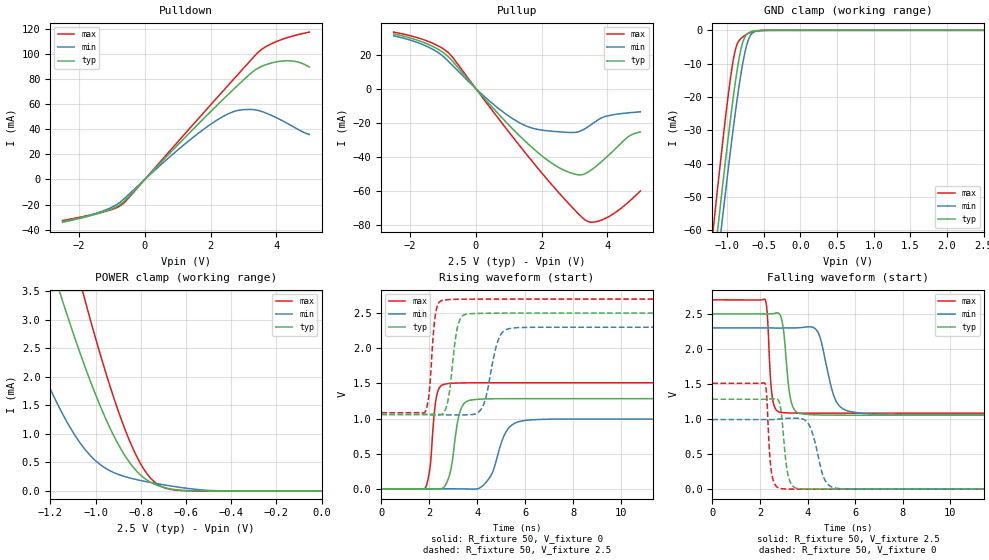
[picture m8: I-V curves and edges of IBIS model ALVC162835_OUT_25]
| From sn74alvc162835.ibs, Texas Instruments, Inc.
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[Model]   ALVC162835_OUT_25
Model_type  3-state
Enable   Active-Low
Vref =   0
Rref =   500
Cref =   30p
Vmeas =   1.25
| variable   typ   min   max
C_comp   5.96pF   4.97pF   7.35pF
| C_pullup   4.89pF   3.51pF   7.52pF
| C_pulldown   4.20pF   3.24pF   5.52pF
| C_tri-state   5.96pF   4.97pF   7.35pF
[Temperature Range]   40   100   -40
| Ambient temperature   25   85   -40
[Voltage range]   2.5   2.3   2.7
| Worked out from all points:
|   slope of the pulldown table from 0 to 0.375 V, typ, clamps not added: 36.2 ohm
|   slope of the pullup table from 0 to 0.375 V, typ, clamps not added: 45.2 ohm
|   GND clamp passes 1 mA (typ) near -0.72 V on its own axis
|   POWER clamp passes 1 mA (typ) near -0.92 V on its own axis
|   rising waveform, R_fixture 50, V_fixture 0: 20-80 % time 338ps typ, 590ps min, 223ps max; typ from 0 V to 1.28 V
|   falling waveform, R_fixture 50, V_fixture 2.5: 20-80 % time 247ps typ, 517ps min, 155ps max; typ from 2.5 V to 1.05 V
|   rising waveform, R_fixture 50, V_fixture 2.5: 20-80 % time 301ps typ, 445ps min, 210ps max; typ from 1.05 V to 2.5 V
|   falling waveform, R_fixture 50, V_fixture 0: 20-80 % time 232ps typ, 435ps min, 156ps max; typ from 1.28 V to 0 V
[GND Clamp]
| ALVC162835_OUT_25
|   Voltage   I(typ)   I(min)   I(max)
-2.5V     -354mA     -357.6mA   -347mA
-1.185V   -71.45mA   -80.34mA   -58.91mA
-1.115V   -57.37mA   -66.56mA   -44.57mA
-1.07V    -48.5mA    -57.85mA   -35.6mA
-960mV    -27.82mA   -37.35mA   -15.45mA
-890mV    -16.04mA   -25.23mA   -6.187mA
-795mV    -4.345mA   -11.06mA   -2.142mA
-740mV    -1.47mA    -5.11mA    -1.307mA
-695mV    -630.7uA   -2.132mA   -797.9uA
-630mV    -200.4uA   -456.3uA   -324.8uA
-500mV    -17.28uA   -21.89uA   -36.4uA
2.5V      1.001nA    1.193nA    10.64nA
[POWER Clamp]
| ALVC162835_OUT_25
|   Voltage   I(typ)   I(min)   I(max)
-2.5V     26.37mA    19.82mA    32.52mA
-1.365V   6.296mA    3.396mA    8.658mA
-1.24V    4.544mA    2.142mA    6.443mA
-1.15V    3.382mA    1.382mA    4.943mA
-1.055V   2.267mA    769.9uA    3.469mA
-1.04V    2.104mA    695.6uA    3.248mA
-960mV    1.31mA     407.9uA    2.141mA
-870mV    618.2uA    250.8uA    1.082mA
-800mV    276.4uA    182.6uA    471.2uA
-740mV    119.3uA    136.4uA    160.3uA
-625mV    13.01uA    61.53uA    7.72uA
-31.15fV  1.001nA    34.52pA    10.39nA
[Pulldown]
| ALVC162835_OUT_25
|   Voltage   I(typ)   I(min)   I(max)
-2.5V     -34.08mA   -33.74mA   -32.77mA
-1.3V     -26.2mA    -25.36mA   -26.18mA
-930mV    -22.61mA   -21.18mA   -23.28mA
-675mV    -18.39mA   -16.42mA   -19.58mA
1.43V     38.99mA    32.72mA    42.58mA
2.155V    58.02mA    46.61mA    63.93mA
2.685V    71.48mA    53.87mA    79.42mA
3.325V    86.63mA    55.53mA    97.95mA
3.53V     89.75mA    54.28mA    103.2mA
3.79V     92.31mA    51.7mA     107.3mA
4.465V    94.38mA    42.67mA    114mA
5V        89.53mA    35.8mA     117.3mA
[Pullup]
| ALVC162835_OUT_25
|   Voltage   I(typ)   I(min)   I(max)
-2.5V     32.2mA     31.07mA    33.27mA
-1.44V    25.97mA    24.4mA     27.73mA
-805mV    18.18mA    15.44mA    20.55mA
360mV     -7.964mA   -6.371mA   -9.294mA
1.22V     -25.71mA   -18.89mA   -30.9mA
1.815V    -36.47mA   -23.73mA   -45.21mA
2.78V     -48.82mA   -25.73mA   -66.79mA
3.21V     -50.68mA   -24.67mA   -75.39mA
3.61V     -46.35mA   -19.73mA   -78.45mA
4.07V     -38.54mA   -15.73mA   -74.97mA
4.605V    -28.69mA   -14.29mA   -67.32mA
5V        -25.5mA    -13.65mA   -60.21mA
[Ramp]
| ALVC162835_OUT_25
| variable   typ   min   max
dV/dt_r   0.77/3.48E-10   0.60/6.00E-10   0.91/2.27E-10
dV/dt_f   0.88/2.54E-10   0.75/5.29E-10   0.98/1.58E-10
R_load = 50
[Rising Waveform]
| ALVC162835_OUT_25
R_fixture =   50
C_fixture =   0
L_fixture =   0
V_fixture =   0
V_fixture_min = 0
V_fixture_max = 0
|   Time   V(typ)   V(min)   V(max)
0s        14.61pV    38.13pV    11.94pV
1.85ns    951.9uV    -48.16uV   19.73mV
2.045ns   338.5uV    127.7uV    340.1mV
2.295ns   -2.423mV   1.118mV    1.3V
2.66ns    44.1mV     332.5uV    1.49V
3.275ns   1.089V     -663.2uV   1.506V
3.715ns   1.261V     -3.717mV   1.508V
4.44ns    1.28V      123.1mV    1.509V
5.885ns   1.283V     967.3mV    1.509V
20ns      1.283V     992.9mV    1.509V
[Falling Waveform]
| ALVC162835_OUT_25
R_fixture =   50
C_fixture =   0
L_fixture =   0
V_fixture =   2.5
V_fixture_min = 2.3
V_fixture_max = 2.7
|   Time   V(typ)   V(min)   V(max)
0s        2.5V       2.3V       2.7V
2.21ns    2.499V     2.3V       2.706V
2.51ns    2.502V     2.3V       1.332V
2.845ns   2.485V     2.299V     1.098V
3.285ns   1.288V     2.3V       1.087V
3.675ns   1.08V      2.304V     1.085V
4.425ns   1.059V     2.245V     1.084V
5.14ns    1.056V     1.298V     1.084V
5.82ns    1.055V     1.105V     1.084V
20ns      1.054V     1.061V     1.084V
[Rising Waveform]
| ALVC162835_OUT_25
R_fixture =   50
C_fixture =   0
L_fixture =   0
V_fixture =   2.5
V_fixture_min = 2.3
V_fixture_max = 2.7
|   Time   V(typ)   V(min)   V(max)
0s        1.054V     1.061V     1.084V
1.845ns   1.054V     1.061V     1.104V
2.26ns    1.049V     1.06V      2.487V
2.555ns   1.067V     1.054V     2.681V
3.18ns    2.304V     1.052V     2.697V
3.52ns    2.484V     1.052V     2.699V
4.225ns   2.498V     1.167V     2.7V
4.86ns    2.499V     2.103V     2.7V
5.36ns    2.5V       2.281V     2.7V
20ns      2.5V       2.3V       2.7V
[Falling Waveform]
| ALVC162835_OUT_25
R_fixture =   50
C_fixture =   0
L_fixture =   0
V_fixture =   0
V_fixture_min = 0
V_fixture_max = 0
|   Time   V(typ)   V(min)   V(max)
0s        1.283V     992.9mV    1.509V
2.2ns     1.283V     992.4mV    1.512V
2.48ns    1.289V     992.5mV    250.4mV
2.85ns    1.188V     1.002V     10.95mV
3.17ns    217.7mV    1.011V     2.1mV
3.585ns   8.766mV    1.012V     580.4uV
4.065ns   1.61mV     913.7mV    168.2uV
4.685ns   416uV      161.2mV    35.81uV
5.185ns   142.1uV    14.78mV    10.75uV
20ns      -3.207nV   4.88nV     -292.2pV
